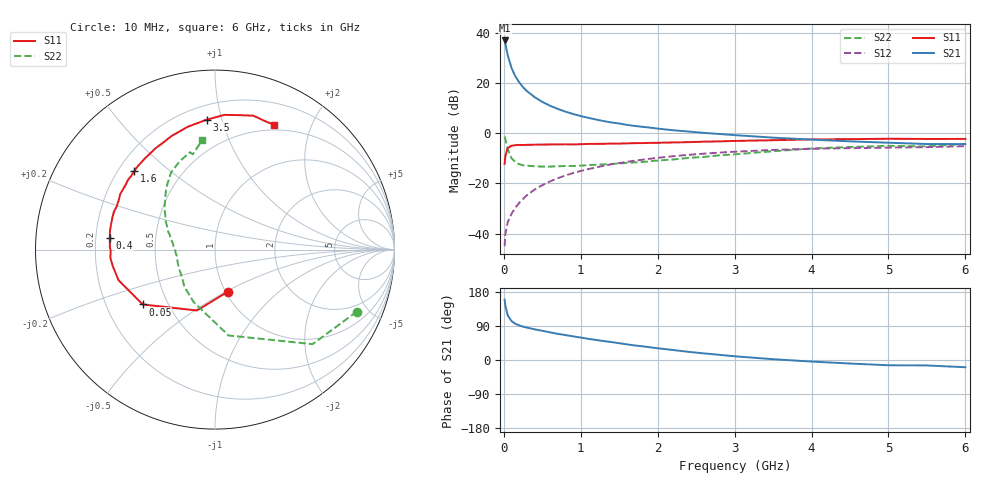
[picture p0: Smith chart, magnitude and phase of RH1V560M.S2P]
! SIEMENS Small Signal Semiconductors
! BFR106
! Si NPN RF Bipolar Junction Transistor in SOT23
! VCE = 1.5 V  IC = 60 mA
! Common Emitter S-Parameters:  August  1996
# GHz  S  MA  R  50
!  f  S11  S21  S12  S22
! GHz  MAG  ANG  MAG  ANG  MAG  ANG  MAG  ANG
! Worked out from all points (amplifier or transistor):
!   36 points, 10 MHz to 6 GHz, reference 50 ohm
!   highest |S21| = 37.0 dB at 10 MHz (marker M1)
!   |S21| within 3 dB of that: start of sweep to 31 MHz
!   unconditionally stable (mu >= 1): 195.3 MHz to 3.072 GHz; 4.355 GHz to end of sweep
!   at 250 MHz: K = 1.05, MAG = 20.8 dB, |S12| = -26.2 dB
!   at 1.4 GHz: K = 1.07, MAG = 6.7 dB, |S12| = -12.4 dB
!   at 6 GHz: K = 1.02, MAG = -0.4 dB, |S12| = -5.2 dB
!   S11 on the Smith chart (normalised r, x): 10 MHz: 1.02, -0.51; 50 MHz: 0.36, -0.30; 400 MHz: 0.26, +0.05; 1.6 GHz: 0.26, +0.38; 3.5 GHz: 0.29, +0.89; 6 GHz: 0.44, +1.49
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0.01  0.2454 -73.3  70.62 159.1  0.0056 75.8  0.8625 -23.6
0.02  0.3539 -106.5  60.51 143.1  0.0098 66.0  0.7569 -44.1
0.05  0.5055 -142.8  35.95 117.8  0.0168 57.8  0.4845 -81.0
0.1  0.5636 -162.4  19.94 102.6  0.0248 62.3  0.3164 -111.9
0.15  0.577 -170.8  13.59 95.5  0.0328 64.8  0.2683 -129.5
0.2  0.5848 -175.5  10.33 91.3  0.0408 68.0  0.2401 -139.8
0.25  0.5812 -179.3  8.252 87.9  0.0491 69.3  0.2294 -148.6
0.3  0.5862 178.5  6.916 85.5  0.0581 70.6  0.2256 -153.7
0.4  0.5897 173.7  5.239 81.0  0.0752 71.1  0.2193 -162.0
0.5  0.5946 169.8  4.208 77.0  0.0922 70.7  0.2162 -167.7
0.6  0.5961 165.7  3.535 72.9  0.1095 70.0  0.216 -171.2
0.7  0.5989 162.5  3.053 69.1  0.1267 68.9  0.2194 -174.3
0.9  0.5982 156.2  2.414 62.4  0.1606 65.9  0.2219 179.3
1.1  0.6119 149.6  2.02 55.8  0.1927 62.6  0.2317 175.6
1.3  0.6152 143.7  1.741 49.9  0.2247 59.1  0.2387 171.0
1.6  0.6278 135.8  1.464 41.3  0.2688 54.0  0.2558 165.5
2.2  0.6545 120.6  1.146 26.3  0.3476 43.4  0.2992 153.5
2.8  0.687 106.7  0.965 13.7  0.4099 33.0  0.3615 141.2
3.5  0.7252 93.7  0.816 2.1  0.4646 22.0  0.4377 128.5
4.5  0.7613 79.7  0.688 -9.3  0.5035 7.9  0.5308 111.6
5.5  0.768 68.5  0.609 -14.4  0.5267 -0.4  0.5451 103.2
6  0.7695 64.7  0.605 -19.1  0.5512 -7.0  0.6141 96.6
